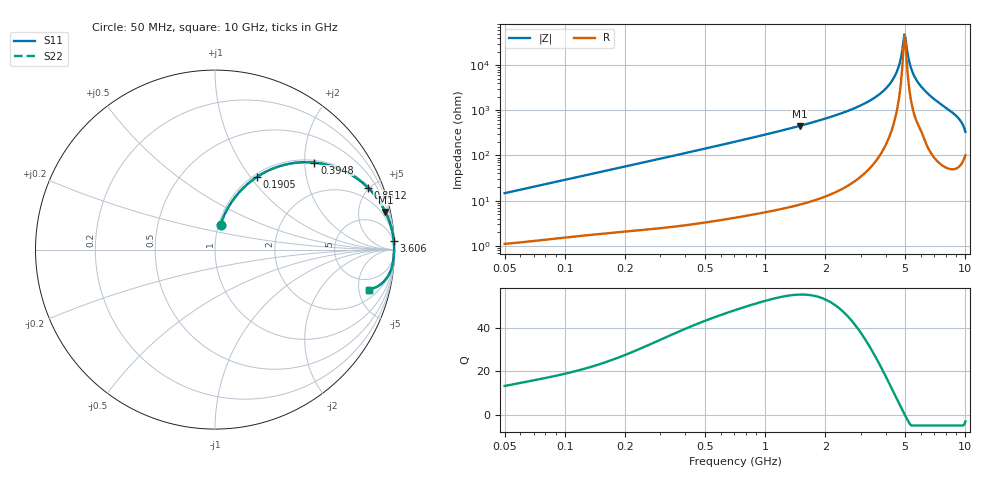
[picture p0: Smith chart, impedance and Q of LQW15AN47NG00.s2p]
!Murata Part Number: LQW15AN47NG00
!These Parameters are Measured in Series Mode Connection
!  o--[Z]--o
!Port1  Port2
!  o-------o
!Freq. Start=50[MHz] Stop=10[GHz], 401[Steps]
# Hz S RI R 50
!Freq.(Hz)	S 11(Real)	S 11(Imag)	S 21(Real)	S 21(Imag)	S 12(Real)	S 12(Imag)	S 22(Real)	S 22(Imag)
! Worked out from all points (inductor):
!   401 points, 50 MHz to 10 GHz, reference 50 ohm
!   read as one part in series: L = 46.2 nH near 51.34 MHz
!   highest Q = 55.5 at 1.485 GHz (marker M1), where L = 48.4 nH
!   self-resonance near 4.956 GHz
!   S11 on the Smith chart (normalised r, x): 50 MHz: 1.02, +0.29; 190.5 MHz: 1.04, +1.08; 394.8 MHz: 1.06, +2.23; 851.2 MHz: 1.10, +4.89; 3.606 GHz: 3, +41; 10 GHz: 3.03, -6.36
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5e7  0.031 0.1397  0.969 -0.1397  0.969 -0.1397  0.031 0.1397
1.214486e8  0.1194 0.3012  0.8806 -0.3012  0.8806 -0.3012  0.1194 0.3012
1.905373e8  0.2351 0.4058  0.7649 -0.4058  0.7649 -0.4058  0.2351 0.4058
2.949953e8  0.4134 0.4781  0.5866 -0.4781  0.5866 -0.4781  0.4134 0.4781
3.947951e8  0.5539 0.4846  0.4461 -0.4846  0.4461 -0.4846  0.5539 0.4846
7.071068e8  0.7978 0.3914  0.2022 -0.3914  0.2022 -0.3914  0.7978 0.3914
8.511793e8  0.8519 0.3455  0.1481 -0.3455  0.1481 -0.3455  0.8519 0.3455
1.484667e9  0.9498 0.2096  0.0502 -0.2096  0.0502 -0.2096  0.9498 0.2096
1.717543e9  0.9637 0.1783  0.0363 -0.1783  0.0363 -0.1783  0.9637 0.1783
2.694605e9  0.9887 0.0946  0.0113 -0.0946  0.0113 -0.0946  0.9887 0.0946
3.606216e9  0.9957 0.0485  0.00426 -0.0485  0.00426 -0.0485  0.9957 0.0485
4.171863e9  0.9974 0.0266  0.00257 -0.0266  0.00257 -0.0266  0.9974 0.0266
4.516952e9  0.9979 0.0147  0.0021 -0.0147  0.0021 -0.0147  0.9979 0.0147
4.700058e9  0.998 0.00869  0.00199 -0.00869  0.00199 -0.00869  0.998 0.00869
4.890587e9  0.998 0.00266  0.00197 -0.00266  0.00197 -0.00266  0.998 0.00266
5.021877e9  0.998 -0.00139  0.00201 0.00139  0.00201 0.00139  0.998 -0.00139
5.088839e9  0.998 -0.00343  0.00205 0.00343  0.00205 0.00343  0.998 -0.00343
5.365732e9  0.9976 -0.0117  0.00235 0.0117  0.00235 0.0117  0.9976 -0.0117
5.809576e9  0.9965 -0.0242  0.00345 0.0242  0.00345 0.0242  0.9965 -0.0242
6.720828e9  0.9949 -0.0485  0.0051 0.0485  0.0051 0.0485  0.9949 -0.0485
8.994549e9  0.9743 -0.1277  0.0257 0.1277  0.0257 0.1277  0.9743 -0.1277
1e10  0.8577 -0.2244  0.1423 0.2244  0.1423 0.2244  0.8577 -0.2244
